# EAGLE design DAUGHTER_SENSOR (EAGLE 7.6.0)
DAUGHTER CARD SENSORS

## Sheet 1 of 3: HDK INTERFACE
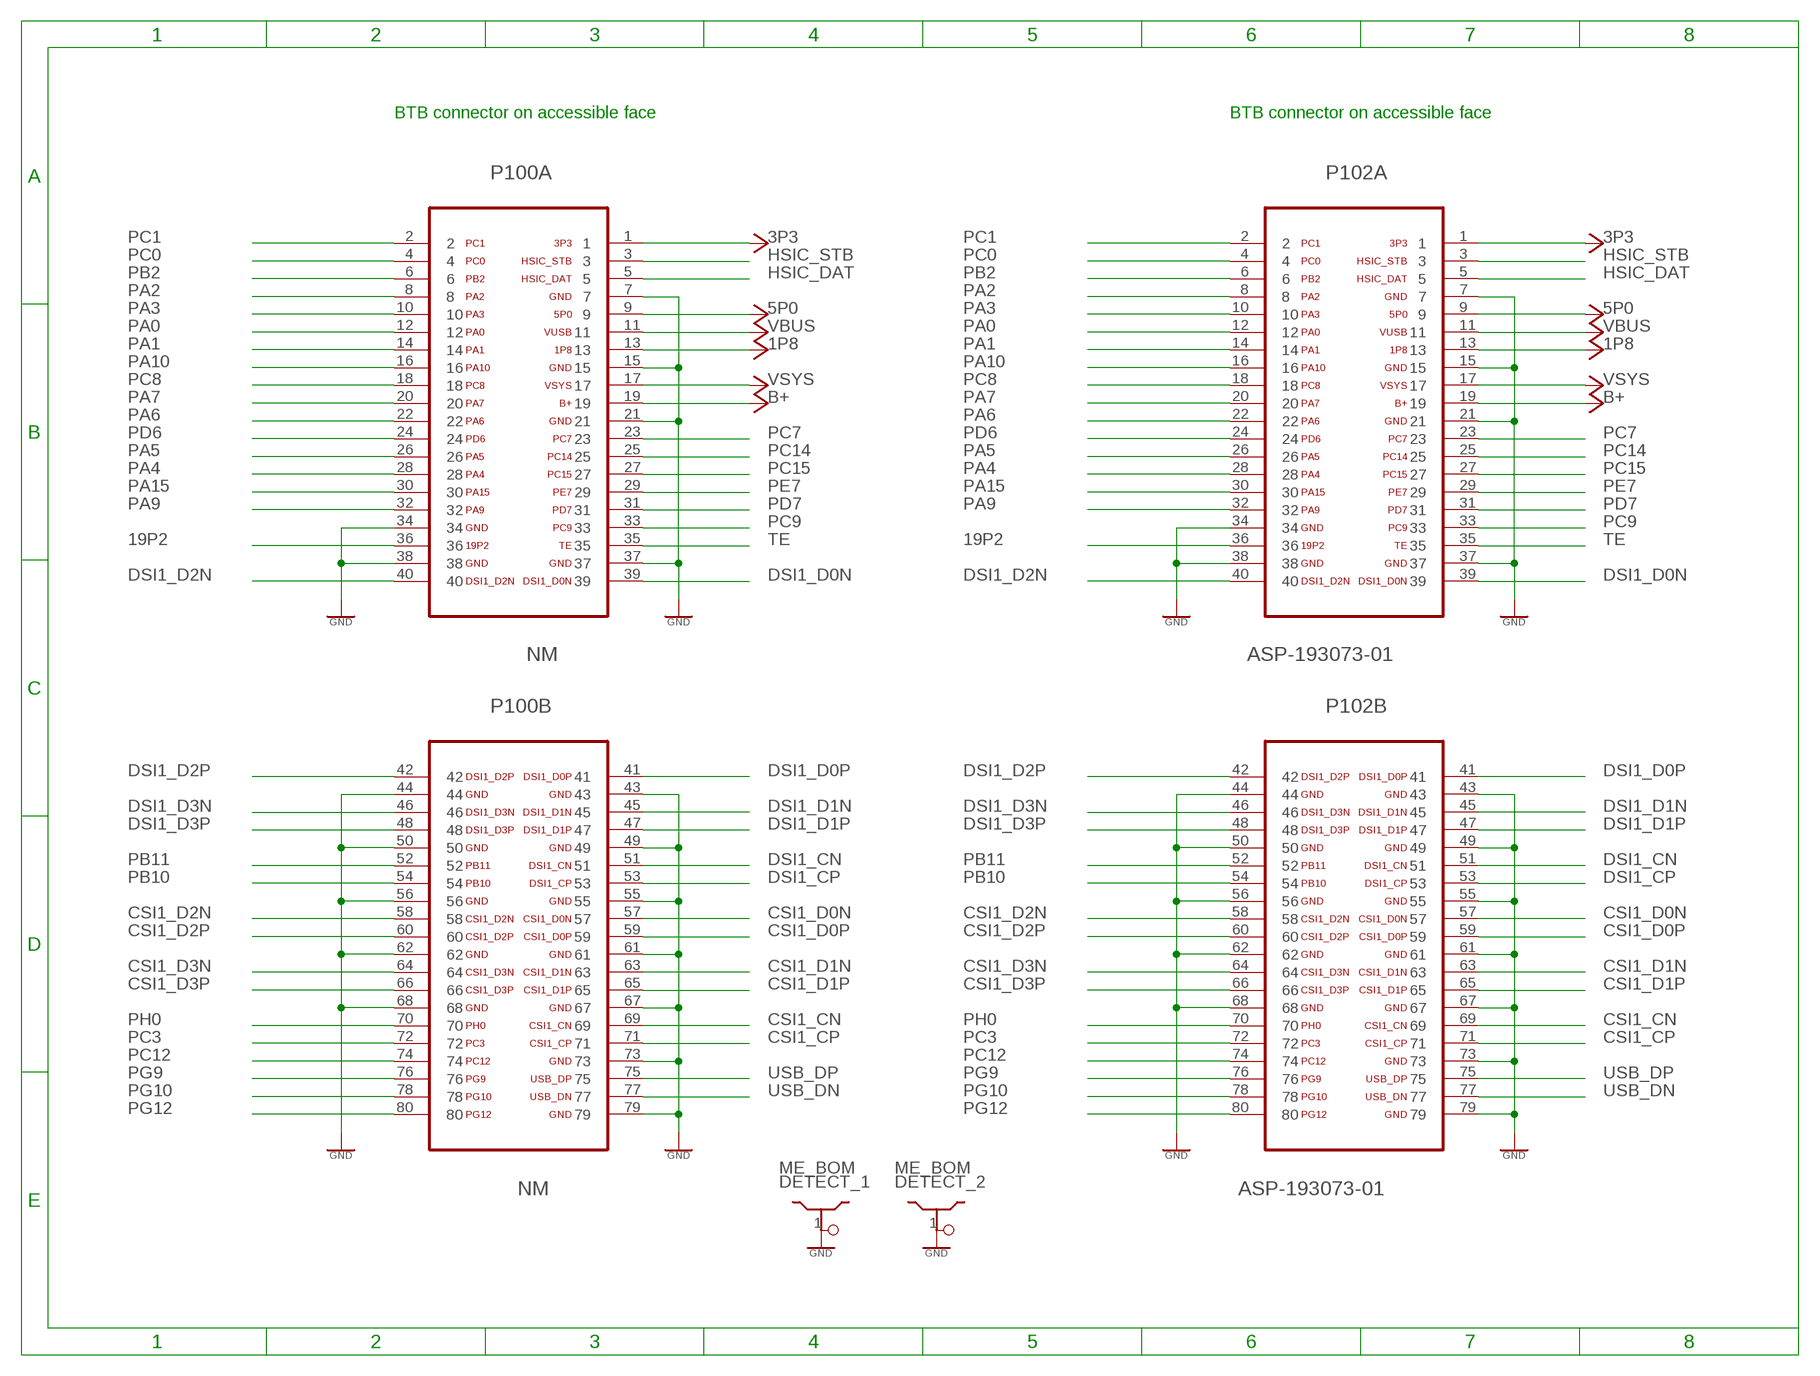
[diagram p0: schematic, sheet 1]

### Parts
DETECT_1  ME_BOM  SHIELDDETECT  [PLUG]
DETECT_2  ME_BOM  SHIELDDETECT  [PLUG]
P100  NM  CLM-140-02-L-D-KGOLD  [CLM-140-02-L-D-K_GOLD]
P102  ASP-193073-01  FTMH-140-02-L-DV-ES-P-TR  [FTMH-140-02-L-DV-ES-P-TR]

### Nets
1P8: P100.13 P102.13 ; also sheet 2,3
3P3: P100.1 P102.1 ; also sheet 2,3
5P0: P100.9 P102.9
19P2: P100.36 P102.36
B+: P100.19 P102.19
CSI1_CN: P100.69 P102.69
CSI1_CP: P100.71 P102.71
CSI1_D0N: P100.57 P102.57
CSI1_D0P: P100.59 P102.59
CSI1_D1N: P100.63 P102.63
CSI1_D1P: P100.65 P102.65
CSI1_D2N: P100.58 P102.58
CSI1_D2P: P100.60 P102.60
CSI1_D3N: P100.64 P102.64
CSI1_D3P: P100.66 P102.66
DSI1_CN: P100.51 P102.51
DSI1_CP: P100.53 P102.53
DSI1_D0N: P100.39 P102.39
DSI1_D0P: P100.41 P102.41
DSI1_D1N: P100.45 P102.45
DSI1_D1P: P100.47 P102.47
DSI1_D2N: P100.40 P102.40
DSI1_D2P: P100.42 P102.42
DSI1_D3N: P100.46 P102.46
DSI1_D3P: P100.48 P102.48
GND: DETECT_1.1 DETECT_2.1 P100.7 P100.15 P100.21 P100.34 P100.37 P100.38 P100.43 P100.44 P100.49 P100.50 P100.55 P100.56 P100.61 P100.62 P100.67 P100.68 P100.73 P100.79 P102.7 P102.15 P102.21 P102.34 P102.37 P102.38 P102.43 P102.44 P102.49 P102.50 P102.55 P102.56 P102.61 P102.62 P102.67 P102.68 P102.73 P102.79 ; also sheet 2,3
HSIC_DAT: P100.5 P102.5
HSIC_STB: P100.3 P102.3
PA0: P100.12 P102.12
PA1: P100.14 P102.14
PA2: P100.8 P102.8
PA3: P100.10 P102.10
PA4: P100.28 P102.28
PA5: P100.26 P102.26
PA6: P100.22 P102.22
PA7: P100.20 P102.20
PA9: P100.32 P102.32
PA10: P100.16 P102.16
PA15: P100.30 P102.30
PB2: P100.6 P102.6
PB10: P100.54 P102.54 ; also sheet 2
PB11: P100.52 P102.52 ; also sheet 2
PC0: P100.4 P102.4 ; also sheet 3
PC1: P100.2 P102.2 ; also sheet 3
PC3: P100.72 P102.72 ; also sheet 3
PC7: P100.23 P102.23
PC8: P100.18 P102.18
PC9: P100.33 P102.33
PC12: P100.74 P102.74
PC14: P100.25 P102.25
PC15: P100.27 P102.27
PD6: P100.24 P102.24
PD7: P100.31 P102.31
PE7: P100.29 P102.29
PG9: P100.76 P102.76 ; also sheet 2
PG10: P100.78 P102.78 ; also sheet 3
PG12: P100.80 P102.80
PH0: P100.70 P102.70
TE: P100.35 P102.35
USB_DN: P100.77 P102.77
USB_DP: P100.75 P102.75
VBUS: P100.11 P102.11
VSYS: P100.17 P102.17

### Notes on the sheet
- BTB connector on accessible face | BTB connector on accessible face

## Sheet 2 of 3: Identification
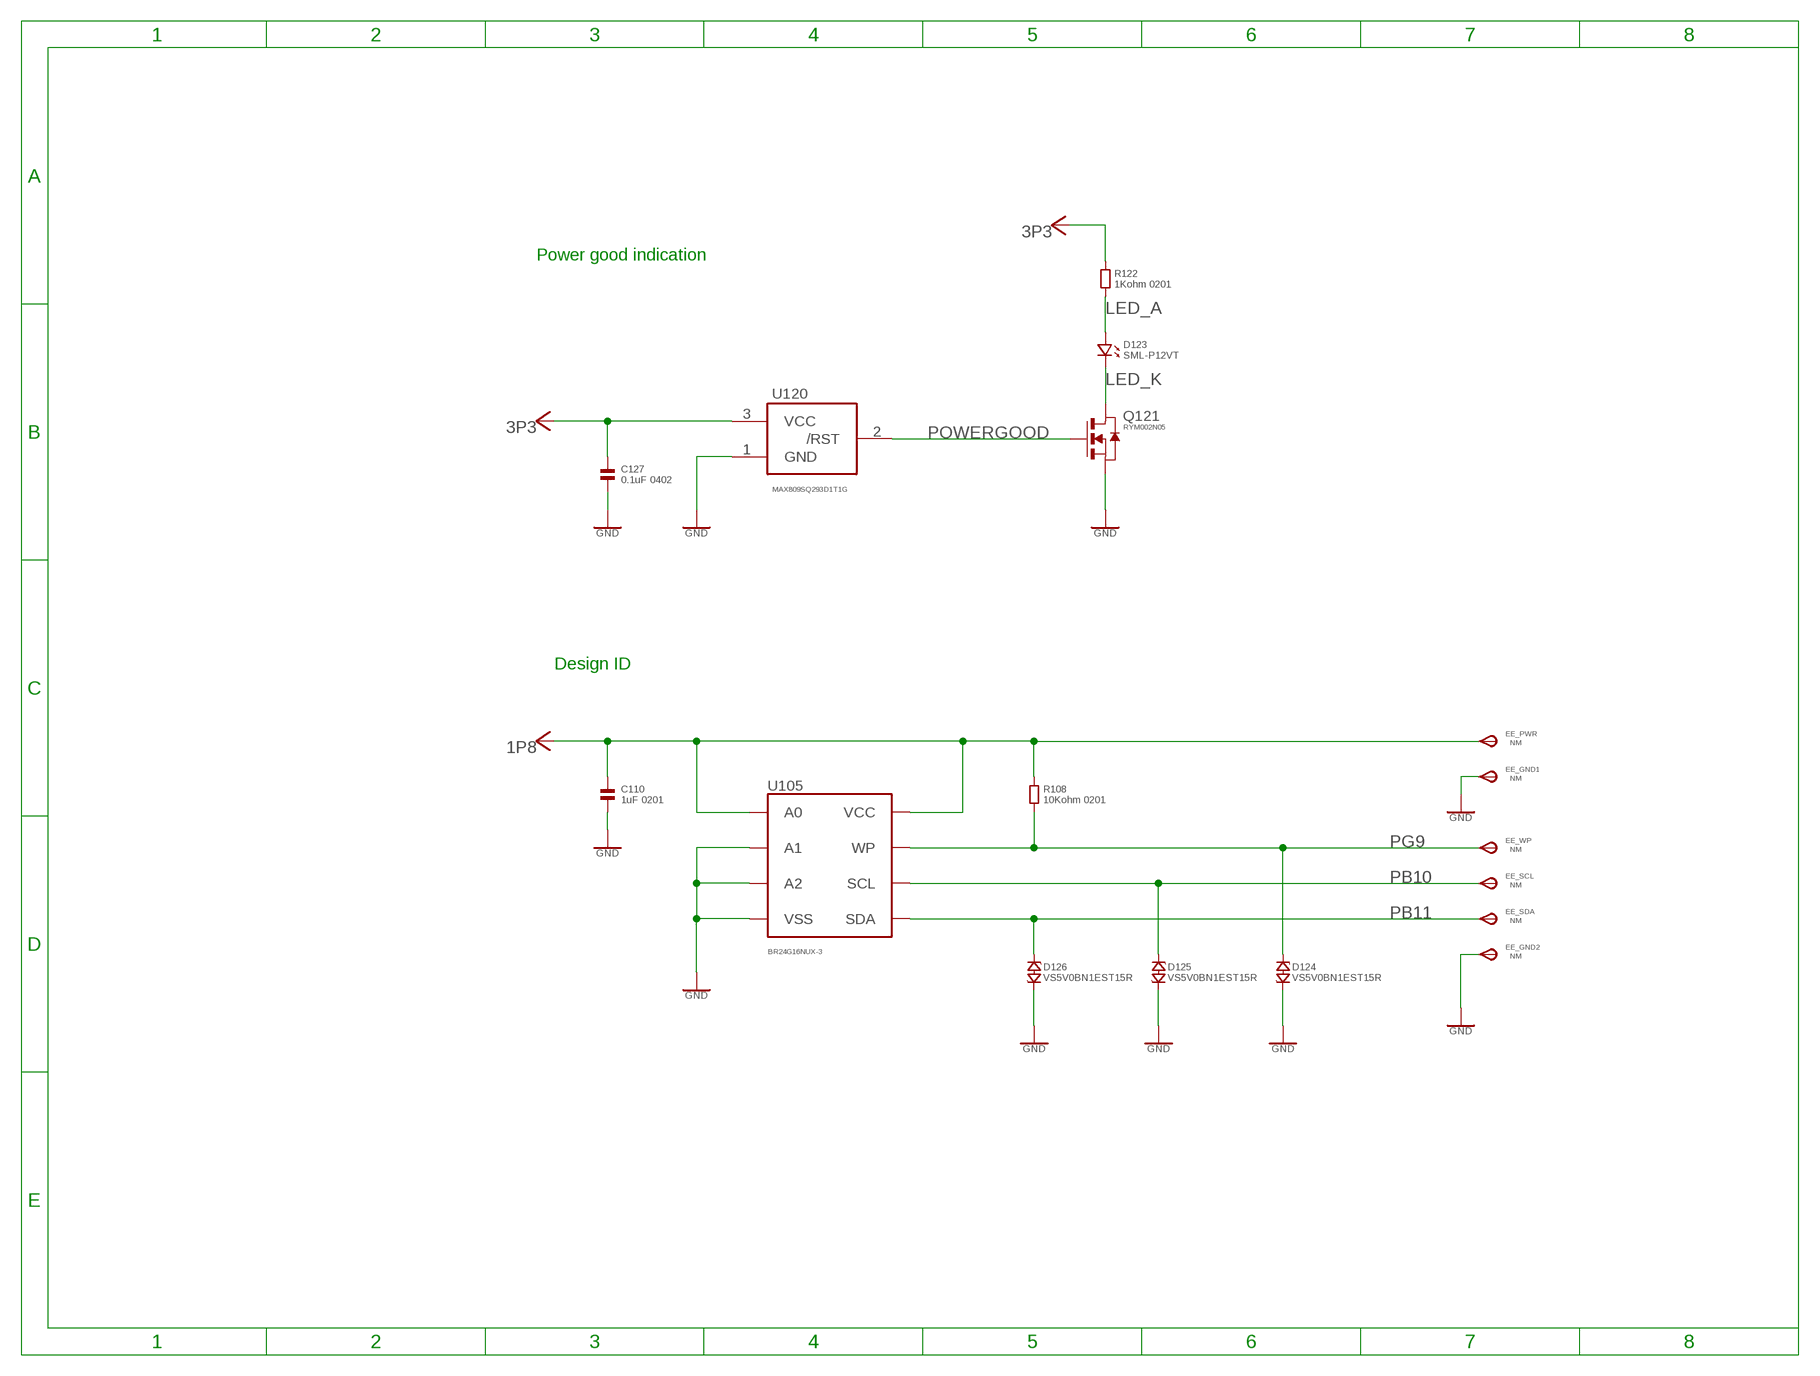
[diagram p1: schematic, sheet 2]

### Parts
C110  1uF 0201  CAPACITOR.0201  [0201]
C127  0.1uF 0402  CAPACITOR.0402  [0402]
D123  SML-P12VT  LED.0503  [0503.LED]
D124  VS5V0BN1EST15R  ESD_VARISTOR.0201  [CHIP_0201]
D125  VS5V0BN1EST15R  ESD_VARISTOR.0201  [CHIP_0201]
D126  VS5V0BN1EST15R  ESD_VARISTOR.0201  [CHIP_0201]
EE_GND1  NM  TPSTP11R  [TP11R]
EE_GND2  NM  TPSTP11R  [TP11R]
EE_PWR  NM  TPSTP11R  [TP11R]
EE_SCL  NM  TPSTP11R  [TP11R]
EE_SDA  NM  TPSTP11R  [TP11R]
EE_WP  NM  TPSTP11R  [TP11R]
Q121  RYM002N05  FET-NRYM002N05  [VMT3]
R108  10Kohm 0201  RESISTOR.0201  [0201]
R122  1Kohm 0201  RESISTOR.0201  [0201]
U105  BR24G16NUX-3  EEPROMDFN8  [DFN-8]
U120  MAX809SQ293D1T1G  MAX809  [SC70-3L]

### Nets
1P8: C110.1 EE_PWR.TP(PP) R108.1 U105.P$1(A0) U105.P$8(VCC) ; also sheet 1,3
3P3: C127.1 R122.1 U120.3(VCC) ; also sheet 1,3
GND: C110.2 C127.2 D124.P$2 D125.P$2 D126.P$2 EE_GND1.TP(PP) EE_GND2.TP(PP) Q121.2(S) U105.P$2(A1) U105.P$3(A2) U105.P$4(VSS) U105.P$9(VSS) U120.1(GND) ; also sheet 1,3
LED_A: D123.P$1 R122.2
LED_K: D123.P$2 Q121.3(D)
PB10: D125.P$1 EE_SCL.TP(PP) U105.P$6(SCL) ; also sheet 1
PB11: D126.P$1 EE_SDA.TP(PP) U105.P$5(SDA) ; also sheet 1
PG9: D124.P$1 EE_WP.TP(PP) R108.2 U105.P$7(WP) ; also sheet 1
POWERGOOD: Q121.1(G) U120.2(/RST)

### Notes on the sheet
- Power good indication
- Design ID

## Sheet 3 of 3: SENSOR
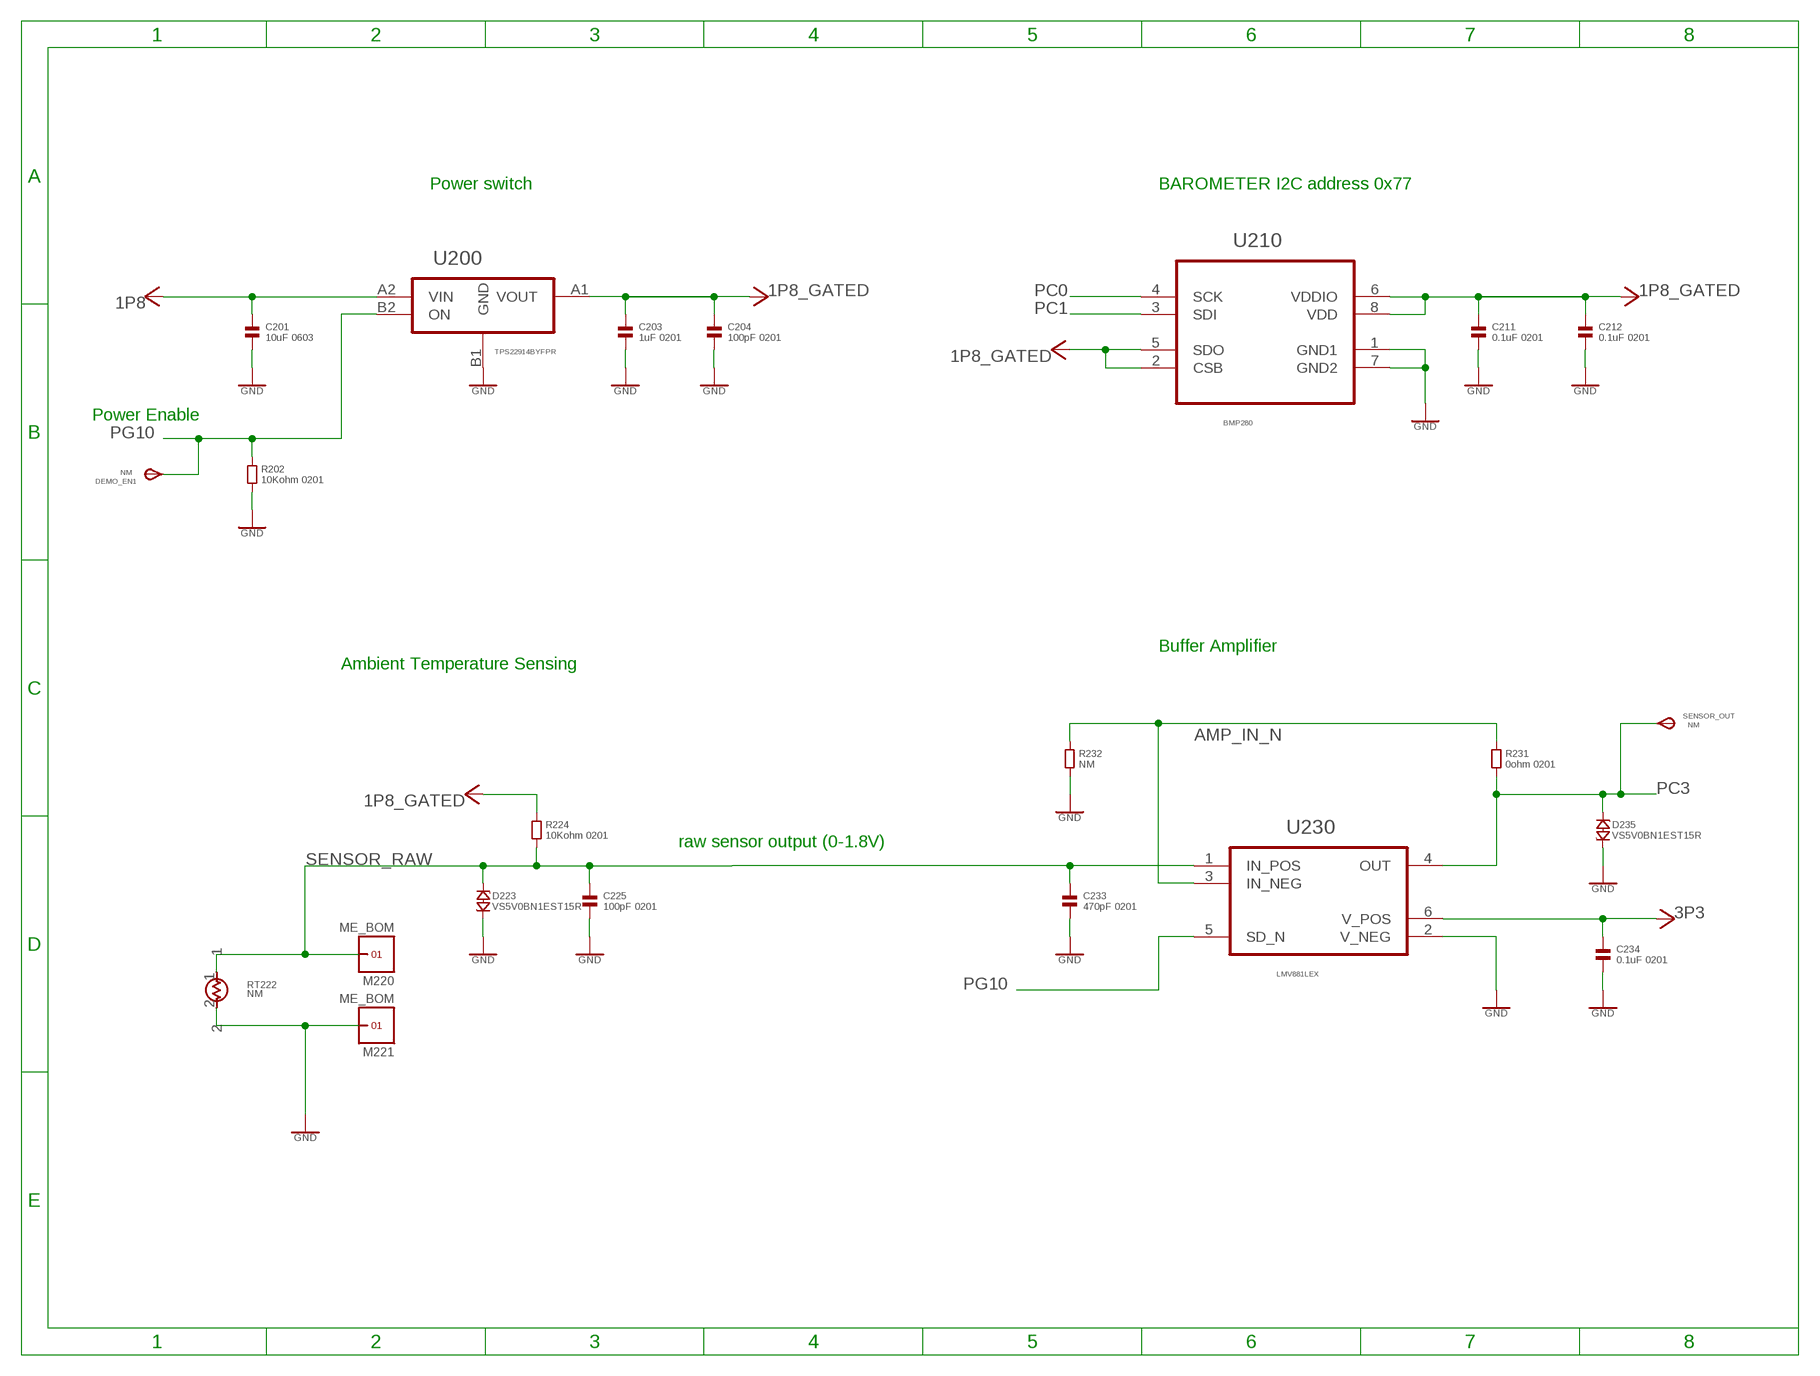
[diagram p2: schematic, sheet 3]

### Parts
C201  10uF 0603  CAPACITOR.0603  [0603]
C203  1uF 0201  CAPACITOR.0201  [0201]
C204  100pF 0201  CAPACITOR.0201  [0201]
C211  0.1uF 0201  CAPACITOR.0201  [0201]
C212  0.1uF 0201  CAPACITOR.0201  [0201]
C225  100pF 0201  CAPACITOR.0201  [0201]
C233  470pF 0201  CAPACITOR.0201  [0201]
C234  0.1uF 0201  CAPACITOR.0201  [0201]
D223  VS5V0BN1EST15R  ESD_VARISTOR.0201  [CHIP_0201]
D235  VS5V0BN1EST15R  ESD_VARISTOR.0201  [CHIP_0201]
DEMO_EN1  NM  TPSTP11R  [TP11R]
M220  ME_BOM  UNVERSA_CONTACT  [UNIVERSAL_CONTACT]
M221  ME_BOM  UNVERSA_CONTACT  [UNIVERSAL_CONTACT]
R202  10Kohm 0201  RESISTOR.0201  [0201]
R224  10Kohm 0201  RESISTOR.0201  [0201]
R231  0ohm 0201  RESISTOR.0201  [0201]
R232  NM  RESISTOR.0201  [0201]
RT222  NM  THERMISTOR  [0201]
SENSOR_OUT  NM  TPSTP11R  [TP11R]
U200  TPS22914BYFPR  [BGA0_75SQ_PS0_4_P4]
U210  BMP280  [LGA2X2_5PS0_65_P8]
U230  LMV881LEX  [DFN1_5X1PS0_5P6]

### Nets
1P8: C201.1 U200.A2(VIN) ; also sheet 1,2
1P8_GATED: C203.1 C204.1 C211.1 C212.1 R224.1 U200.A1(VOUT) U210.2(CSB) U210.5(SDO) U210.6(VDDIO) U210.8(VDD)
3P3: C234.1 U230.6(V_POS) ; also sheet 1,2
AMP_IN_N: R231.1 R232.1 U230.3(IN_NEG)
GND: C201.2 C203.2 C204.2 C211.2 C212.2 C225.2 C233.2 C234.2 D223.P$2 D235.P$2 M221.G1 R202.2 R232.2 RT222.2 U200.B1(GND) U210.1(GND1) U210.7(GND2) U230.2(V_NEG) ; also sheet 1,2
PC0: U210.4(SCK) ; also sheet 1
PC1: U210.3(SDI) ; also sheet 1
PC3: D235.P$1 R231.2 SENSOR_OUT.TP(PP) U230.4(OUT) ; also sheet 1
PG10: DEMO_EN1.TP(PP) R202.1 U200.B2(ON) U230.5(SD_N) ; also sheet 1
SENSOR_RAW: C225.1 C233.1 D223.P$1 M220.G1 R224.2 RT222.1 U230.1(IN_POS)

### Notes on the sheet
- Power switch | BAROMETER I2C address 0x77
- Power Enable
- Buffer Amplifier
- Ambient Temperature Sensing
- raw sensor output (0-1.8V)

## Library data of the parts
C110 C127 C201 C203 C204 C211 C212 C225 C233 C234 = MOTO_LIB:CAPACITOR: Ceramic Capacitor, Generic
D123 = MOTO_LIB:LED: LED GENERIC, single, 2 pin; MPN: SML-P12VT; SUPPLIER: ROHM
D124-D126 D223 D235 = MOTO_LIB:ESD_VARISTOR: GENERIC varistor,single, 2 pin; MPN: VS5V0BN1EST15R; SUPPLIER: ROHM
DEMO_EN1 EE_GND1 EE_GND2 EE_PWR EE_SCL EE_SDA EE_WP SENSOR_OUT = MOTO_LIB:TPS: TEST Point, 1mm diameter, gold
DETECT_1 DETECT_2 = MOTO_LIB:SHIELD: Shield, Custom; MPN: refer to ME BOM; SUPPLIER: ref to ME BOM
M220 M221 = MOTO_LIB:UNVERSA_CONTACT: Universal contact, Generic; MPN: refer to ME BOM; SUPPLIER: ref to ME BOM
P100 = MOTO_LIB:CLM-140-02-L-D-K: MICRO SOCKET, 1.0MM pitch, SMD, 2X40WAY, Female; MPN: CLM-140-02-L-D-K; SUPPLIER: SAMTEC
P102 = MOTO_LIB:FTMH-140-02-L-DV-ES-P-TR: MICRO SOCKET, 1.0MM, SMD, 2X40WAY, MALE; MPN: ASP-193073-01; SUPPLIER: SAMTEC
Q121 = MOTO_LIB:FET-N: Generic NMOS FET; MPN: RYM002N05; SUPPLIER: ROHM
R108 R122 R202 R224 R231 R232 = MOTO_LIB:RESISTOR: Resistor - Generic
RT222 = MOTO_LIB:THERMISTOR: Thmistor, NTC 10Khm 3%, 0201; MPN: NCP03XV103XV103E05RL/NTCG0603UH103HT; SUPPLIER: MURARA/TDK
U105 = MOTO_LIB:EEPROM: I2C EE PROM, 8 pin; MPN: BR24G16NUX-3; SUPPLIER: ROHM
U120 = MOTO_LIB:MAX809: 3-Pin Microprocessor Reset Circuit; MPN: MAX809SQ293D1T1; SUPPLIER: ON-SEMI
U200 = MOTO_LIB:TPS22914BYFPR: 5V load switch; MPN: TPS22914BYFPR; SUPPLIER: TI
U210 = MOTO_LIB:BMP280: BAROMETER BMP280; MPN: BMP280; SUPPLIER: BOSCH
U230 = MOTO_LIB:LMV881LEX: LOW NOISE OPAMP with Shutdown.; MPN: LMV881LEX; SUPPLIER: TI

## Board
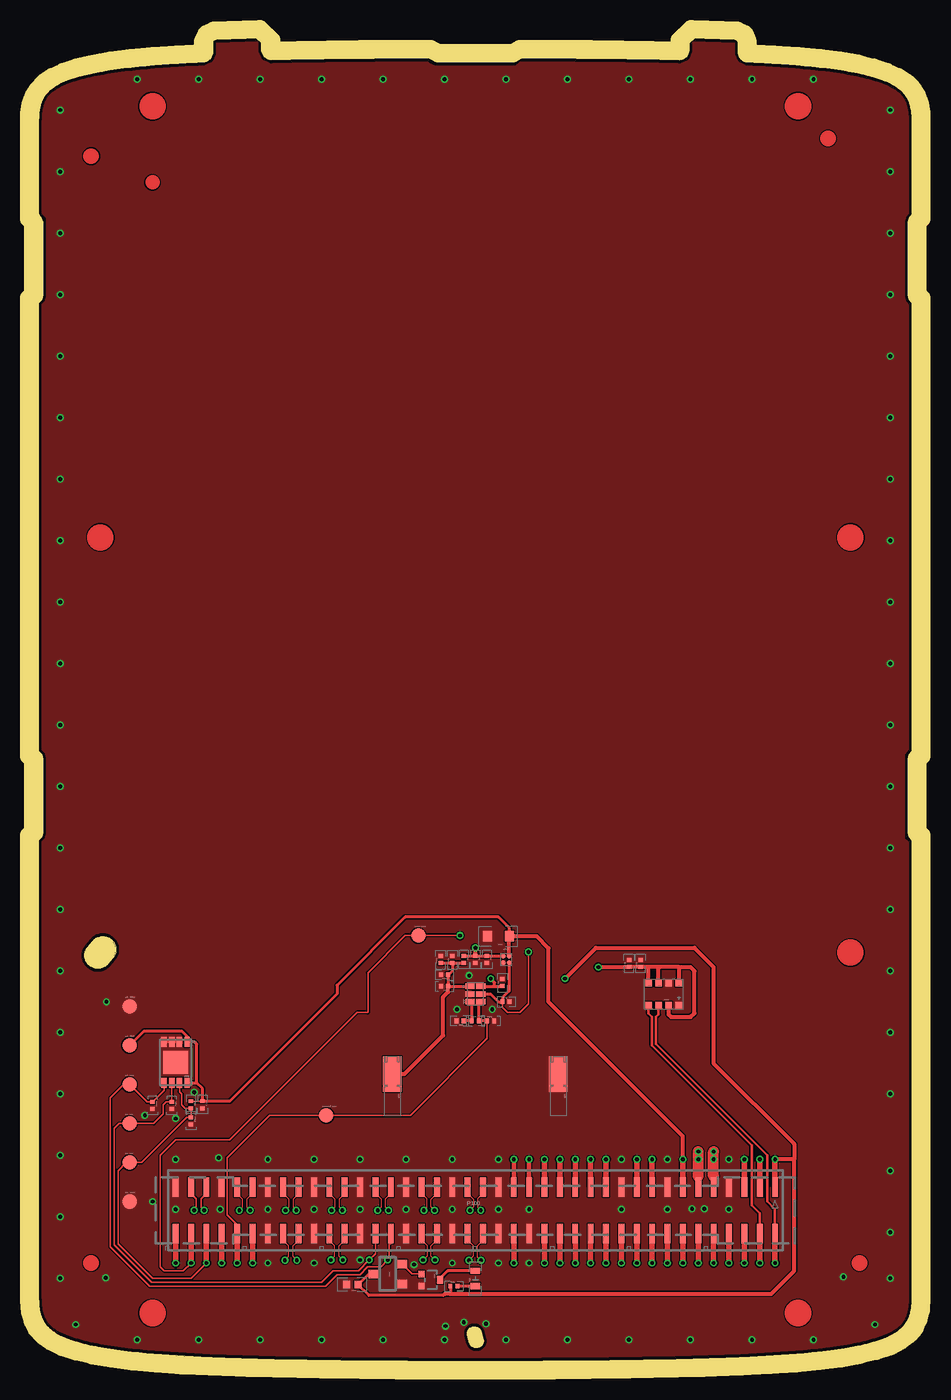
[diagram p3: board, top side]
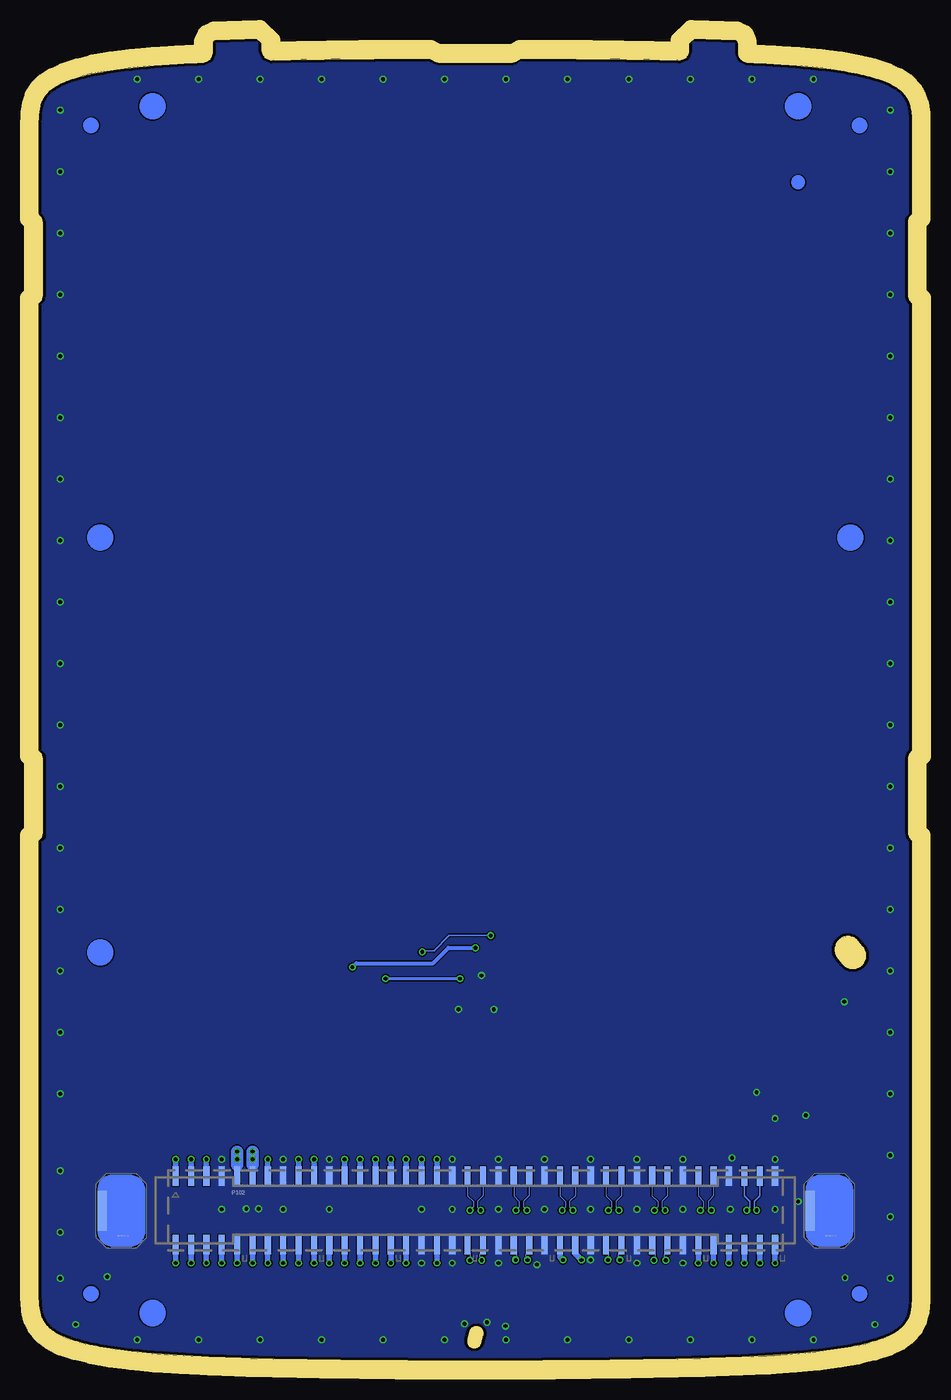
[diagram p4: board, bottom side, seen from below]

Size 56.85 x 86.03 mm. Coordinates in mm from the lower left corner, seen from the top.
Outline: 357 segments
Copper layers (1*2*15*16): Top 0.02mm / dielectric 0.045mm / Route2 0.016mm / dielectric 0.711mm / Route15 0.016mm / dielectric 0.045mm / Bottom 0.02mm
Design rules "constraint": minimum track width 0.08mm, minimum drill 0.25mm, track to track 0.08mm, track to pad 0.08mm, pad to pad 0.08mm, via to via 0.08mm, smd to smd 0.08mm, copper to edge 0.2mm, drill to drill 0.2mm, minimum pad ring 0.1mm, minimum via ring 0.1mm, stop-mask expansion 0mil, vias tented up to drill 0.25mm, thermal gap 0mil
Milling: 125 lines

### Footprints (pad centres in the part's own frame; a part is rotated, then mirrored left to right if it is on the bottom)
0201 = smd 0.25 x 0.3: 1 -0.23,0; 2 0.23,0
0402 = smd 0.45 x 0.5: 1 -0.37,0; 2 0.37,0
0603 = smd 0.58 x 0.68: 1 -0.71,0; 2 0.71,0
0503.LED = smd 0.4 x 0.6: P$1 -0.495,0; P$2 0.495,0
CHIP_0201 = smd 0.25 x 0.3: P$1 -0.23,0; P$2 0.23,0
TP11R = smd 0.95 x 0.95: TP 0,0
PLUG = smd 0.6 x 2.6: 1 -1.25,0
UNIVERSAL_CONTACT = smd 2.3 x 1.2: G1 -0.8,0
CLM-140-02-L-D-K_GOLD = smd 0.38 x 1.27: 1 19.5,1.52; 2 19.5,-1.52; 3 18.5,1.52; 4 18.5,-1.52; 5 17.5,1.52; 6 17.5,-1.52; 7 16.5,1.52; 8 16.5,-1.52; 9 15.5,1.52; 10 15.5,-1.52; 11 14.5,1.52; 12 14.5,-1.52; 13 13.5,1.52; 14 13.5,-1.52; 15 12.5,1.52; 16 12.5,-1.52; 17 11.5,1.52; 18 11.5,-1.52; 19 10.5,1.52; 20 10.5,-1.52; 21 9.5,1.52; 22 9.5,-1.52; 23 8.5,1.52; 24 8.5,-1.52; 25 7.5,1.52; 26 7.5,-1.52; 27 6.5,1.52; 28 6.5,-1.52; 29 5.5,1.52; 30 5.5,-1.52; 31 4.5,1.52; 32 4.5,-1.52; 33 3.5,1.52; 34 3.5,-1.52; 35 2.5,1.52; 36 2.5,-1.52; 37 1.5,1.52; 38 1.5,-1.52; 39 0.5,1.52; 40 0.5,-1.52; 41 -0.5,1.52; 42 -0.5,-1.52; 43 -1.5,1.52; 44 -1.5,-1.52; 45 -2.5,1.52; 46 -2.5,-1.52; 47 -3.5,1.52; 48 -3.5,-1.52; 49 -4.5,1.52; 50 -4.5,-1.52; 51 -5.5,1.52; 52 -5.5,-1.52; 53 -6.5,1.52; 54 -6.5,-1.52; 55 -7.5,1.52; 56 -7.5,-1.52; 57 -8.5,1.52; 58 -8.5,-1.52; 59 -9.5,1.52; 60 -9.5,-1.52; 61 -10.5,1.52; 62 -10.5,-1.52; 63 -11.5,1.52; 64 -11.5,-1.52; 65 -12.5,1.52; 66 -12.5,-1.52; 67 -13.5,1.52; 68 -13.5,-1.52; 69 -14.5,1.52; 70 -14.5,-1.52; 71 -15.5,1.52; 72 -15.5,-1.52; 73 -16.5,1.52; 74 -16.5,-1.52; 75 -17.5,1.52; 76 -17.5,-1.52; 77 -18.5,1.52; 78 -18.5,-1.52; 79 -19.5,1.52; 80 -19.5,-1.52
FTMH-140-02-L-DV-ES-P-TR = smd 0.4 x 1.263: 1 -19.5,2.223; 2 -19.5,-2.223; 3 -18.5,2.223; 4 -18.5,-2.223; 5 -17.5,2.223; 6 -17.5,-2.223; 7 -16.5,2.223; 8 -16.5,-2.223; 9 -15.5,2.223; 10 -15.5,-2.223; 11 -14.5,2.223; 12 -14.5,-2.223; 13 -13.5,2.223; 14 -13.5,-2.223; 15 -12.5,2.223; 16 -12.5,-2.223; 17 -11.5,2.223; 18 -11.5,-2.223; 19 -10.5,2.223; 20 -10.5,-2.223; 21 -9.5,2.223; 22 -9.5,-2.223; 23 -8.5,2.223; 24 -8.5,-2.223; 25 -7.5,2.223; 26 -7.5,-2.223; 27 -6.5,2.223; 28 -6.5,-2.223; 29 -5.5,2.223; 30 -5.5,-2.223; 31 -4.5,2.223; 32 -4.5,-2.223; 33 -3.5,2.223; 34 -3.5,-2.223; 35 -2.5,2.223; 36 -2.5,-2.223; 37 -1.5,2.223; 38 -1.5,-2.223; 39 -0.5,2.223; 40 -0.5,-2.223; 41 0.5,2.223; 42 0.5,-2.223; 43 1.5,2.223; 44 1.5,-2.223; 45 2.5,2.223; 46 2.5,-2.223; 47 3.5,2.223; 48 3.5,-2.223; 49 4.5,2.223; 50 4.5,-2.223; 51 5.5,2.223; 52 5.5,-2.223; 53 6.5,2.223; 54 6.5,-2.223; 55 7.5,2.223; 56 7.5,-2.223; 57 8.5,2.223; 58 8.5,-2.223; 59 9.5,2.223; 60 9.5,-2.223; 61 10.5,2.223; 62 10.5,-2.223; 63 11.5,2.223; 64 11.5,-2.223; 65 12.5,2.223; 66 12.5,-2.223; 67 13.5,2.223; 68 13.5,-2.223; 69 14.5,2.223; 70 14.5,-2.223; 71 15.5,2.223; 72 15.5,-2.223; 73 16.5,2.223; 74 16.5,-2.223; 75 17.5,2.223; 76 17.5,-2.223; 77 18.5,2.223; 78 18.5,-2.223; 79 19.5,2.223; 80 19.5,-2.223
VMT3 = smd 0.42 x 0.4: 1 -0.4,-0.6; 2 0.4,-0.6 | smd 0.52 x 0.4: 3 0,0.6
DFN-8 = smd 0.35 x 0.65: P$1 -0.75,-1.325; P$2 -0.25,-1.325; P$3 0.25,-1.325; P$4 0.75,-1.325; P$5 0.75,1.325; P$6 0.25,1.325; P$7 -0.25,1.325; P$8 -0.75,1.325 | smd 1.6 x 1.5: P$9 0,0
SC70-3L = smd 0.55 x 0.63: 1 -0.65,-0.94; 3 0,0.94 | smd 0.555 x 0.63: 2 0.65,-0.94
BGA0_75SQ_PS0_4_P4 = smd 0.32 x 0.32: A1 -0.2,0.2; A2 0.2,0.2; B1 -0.2,-0.2; B2 0.2,-0.2
LGA2X2_5PS0_65_P8 = smd 0.45 x 0.45: 1 -0.975,0.725; 2 -0.325,0.725; 3 0.325,0.725; 4 0.975,0.725; 5 0.975,-0.725; 6 0.325,-0.725; 7 -0.325,-0.725; 8 -0.975,-0.725
DFN1_5X1PS0_5P6 = smd 0.35 x 0.6: 1 0.5,0.35; 2 0,0.35; 3 -0.5,0.35; 4 -0.5,-0.35; 5 0,-0.35; 6 0.5,-0.35

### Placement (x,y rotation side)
C110  10.67,16.67 270 top
C127  20.42,4.97 180 top
C201  29.92,27.62 180 top
C203  29.17,26.12 270 top
C204  28.42,26.12 270 top
C211  39.17,25.87 90 top
C212  38.42,25.87 90 top
C225  26.17,26.12 90 top
C233  26.92,26.12 90 top
C234  30.17,24.62 90 top
D123  28.42,5.37 90 top
D124  9.92,15.62 270 top
D125  8.67,16.62 270 top
D126  7.42,16.62 270 top
D223  26.42,24.37 180 top
D235  29.42,22.12 0 top
DEMO_EN1  24.72,27.67 0 top
DETECT_1  51.45,9.77 0 bottom
DETECT_2  5.39,9.77 0 bottom
EE_GND1  5.92,10.37 0 top
EE_GND2  5.92,23.07 0 top
EE_PWR  5.92,20.53 0 top
EE_SCL  5.92,15.45 0 top
EE_SDA  5.92,17.99 0 top
EE_WP  5.92,12.91 0 top
M220  23.02,17.87 270 top
M221  33.82,17.87 270 top
P100  28.42,9.8 0 top
P102  28.42,9.8 0 bottom
Q121  25.52,5.27 270 top
R108  9.92,16.67 270 top
R122  27.02,4.87 0 top
R202  30.42,23.37 0 top
R224  27.67,26.12 270 top
R231  28.42,22.12 0 top
R232  27.42,22.12 180 top
RT222  26.42,25.12 180 top
SENSOR_OUT  18.72,15.97 0 top
U105  8.92,19.42 180 top
U120  22.72,5.67 90 top
U200  30.42,26.12 0 top
U210  40.67,23.87 180 top
U230  28.42,23.87 90 top

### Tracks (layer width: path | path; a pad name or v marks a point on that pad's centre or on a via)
1P8  (via drill 0.25)
  Top 0.1: R108.1 C110.1
  Top 0.2: EE_PWR.TP 6.86,21.47 9.32,21.47 9.67,21.12 U105.P$1 10.15,20.75 10.3,20.6 10.3,18.1 | U105.P$8 10.3,18.1 | 10.3,18.1 10.67,17.72 C110.1 12.45,16.9 19.42,23.87 19.42,24.44 23.86,28.87 29.92,28.87 30.63,28.16 C201.1
  Top 0.25: C201.1 32.42,27.62 33.19,26.86 33.19,23.36 41.92,14.62 v41.92,13.12 | U200.A2 C201.1
  Top 0.35: C201.1 | P100.13 v41.92,13.12
  Bottom 0.35: P102.13 v41.92,13.12
1P8_GATED  (via drill 0.25)
  Top 0.2: U200.A1 30.19,26.35 C203.1 C204.1 R224.1
  Top 0.25: C204.1 v28.42,26.87 | v36.42,25.62 38.4,25.62 C212.1 C211.1 39.19,25.62 39.67,25.62 | 41.65,25.62 41.65,24.62 U210.8 | U210.2 41,22.55 41.17,22.37 42.42,22.37 42.67,22.62 42.67,25.37 | 42.67,25.37 42.42,25.62 | 42.42,25.62 42.67,25.37 | 41.65,25.62 41.67,25.62 42.42,25.62 | 41.65,25.62 40.42,25.62 | 40.42,25.62 39.67,25.62 | U210.6 40.35,25.55 40.42,25.62 | U210.5 39.7,25.6 39.67,25.62
  Bottom 0.25: v28.42,26.87 30.17,26.87 31.17,25.87 36.17,25.87 v36.42,25.62
3P3  (via drill 0.25)
  Top 0.2: U230.6 29.67,24.37 | 29.67,24.37 30.15,24.37 C234.1 | 29.67,24.37 29.67,24.62 v29.42,24.87 | U120.3 21.49,5.67 C127.1 21.49,4.27 26.32,4.27 26.42,4.37 | R122.1 26.79,4.37
  Top 0.25: v34.26,24.87 36.26,26.87 42.67,26.87 43.92,25.62 43.92,19.37 49.17,14.12 49.17,13.12 | 49.17,13.12 v47.92,13.12 | 26.42,4.37 26.79,4.37 47.67,4.37 49.17,5.87 49.17,13.12
  Top 0.35: P100.1 v47.92,13.12
  Bottom 0.2: v29.42,24.87 v34.26,24.87
  Bottom 0.35: P102.1 v47.92,13.12
5P0  (via drill 0.25)
  Top 0.25: P100.9 P102.9
  Top 0.7: P102.9 v43.92,13.62
  Bottom 0.4: P102.9 43.92,12.77
  Bottom 0.8: 43.92,12.77 v43.92,13.12 v43.92,13.62
19P2  (via drill 0.25)
  Top 0.35: P100.36 v30.92,6.37
  Bottom 0.35: v30.92,6.37 P102.36
AMP_IN_N
  Top 0.2: R232.1 R231.1 28.19,23.25 U230.3
B+  (via drill 0.25)
  Top 0.35: P100.19 v38.92,13.12
  Bottom 0.35: v38.92,13.12 P102.19
CSI1_CN  (via drill 0.25)
  Top 0.08: P100.69 13.92,10.9 13.57,10.55 13.57,10 v13.77,9.8
  Bottom 0.08: P102.69 13.92,10.75 13.57,10.4 13.57,10 v13.77,9.8
CSI1_CP  (via drill 0.25)
  Top 0.08: P100.71 12.92,10.9 13.29,10.53 13.29,10.02 v13.07,9.8
  Bottom 0.08: P102.71 12.92,10.75 13.27,10.4 13.27,10 v13.07,9.8
CSI1_D0N  (via drill 0.25)
  Top 0.08: P100.57 19.92,10.9 19.55,10.53 19.55,10.02 v19.77,9.8
  Bottom 0.08: P102.57 19.92,10.75 19.57,10.4 19.57,10 v19.77,9.8
CSI1_D0P  (via drill 0.25)
  Top 0.08: P100.59 18.92,10.9 19.27,10.55 19.27,10 v19.07,9.8
  Bottom 0.08: P102.59 18.92,10.75 19.29,10.38 19.29,10.02 v19.07,9.8
CSI1_D1N  (via drill 0.25)
  Top 0.08: P100.63 16.92,10.9 16.55,10.53 16.55,10.02 v16.77,9.8
  Bottom 0.08: P102.63 16.92,10.75 16.55,10.38 16.55,10.02 v16.77,9.8
CSI1_D1P  (via drill 0.25)
  Top 0.08: 15.92,10.9 16.27,10.55 16.27,10 v16.07,9.8
  Top 0.1: P100.65 15.92,10.9
  Bottom 0.08: P102.65 15.92,10.75 16.27,10.4 16.27,10 v16.07,9.8
CSI1_D2N  (via drill 0.25)
  Top 0.08: P100.58 19.92,7.85 19.57,7.5 19.57,6.8 v19.8,6.58
  Bottom 0.08: P102.58 19.92,7.17 19.72,6.97 19.72,6.65 v19.8,6.58
CSI1_D2P  (via drill 0.25)
  Top 0.08: P100.60 18.92,7.85 19.27,7.5 19.27,6.82 v19.03,6.58
  Bottom 0.08: P102.60 18.92,7.15 19.12,6.95 19.12,6.67 v19.03,6.58
CSI1_D3N  (via drill 0.25)
  Top 0.08: P100.64 16.92,7.85 16.57,7.5 16.57,6.8 v16.81,6.57
  Bottom 0.08: P102.64 16.92,7.12 16.72,6.92 16.72,6.65 v16.81,6.57
CSI1_D3P  (via drill 0.25)
  Top 0.08: P100.66 15.92,7.85 16.27,7.5 16.27,6.8 v16.03,6.57
  Bottom 0.08: P102.66 15.92,7.12 16.12,6.92 16.12,6.65 v16.03,6.57
DSI1_CN  (via drill 0.25)
  Top 0.08: 22.92,10.9 22.55,10.53 22.55,10.02 v22.77,9.8
  Top 0.1: P100.51 22.92,10.9
  Bottom 0.08: P102.51 22.92,10.75 22.57,10.4 22.57,10 v22.77,9.8
DSI1_CP  (via drill 0.25)
  Top 0.08: P100.53 21.92,10.9 22.27,10.55 22.27,10 v22.07,9.8
  Bottom 0.08: P102.53 21.92,10.75 22.29,10.39 22.29,10.02 v22.07,9.8
DSI1_D0N  (via drill 0.25)
  Top 0.08: P100.39 28.92,10.9 28.57,10.55 28.57,10 v28.77,9.8
  Bottom 0.08: P102.39 28.92,10.75 28.55,10.38 28.55,10.02 v28.77,9.8
DSI1_D0P  (via drill 0.25)
  Top 0.08: P100.41 27.92,10.9 28.29,10.53 28.29,10.02 v28.07,9.8
  Bottom 0.08: P102.41 27.92,10.75 28.27,10.4 28.27,10 v28.07,9.8
DSI1_D1N  (via drill 0.25)
  Top 0.08: P100.45 25.92,10.9 25.55,10.53 25.55,10.02 v25.77,9.8
  Bottom 0.08: P102.45 25.92,10.75 25.57,10.4 25.57,10 v25.77,9.8
DSI1_D1P  (via drill 0.25)
  Top 0.08: P100.47 24.92,10.9 25.27,10.55 25.27,10 v25.07,9.8
  Bottom 0.08: P102.47 24.92,10.75 25.29,10.38 25.29,10.02 v25.07,9.8
DSI1_D2N  (via drill 0.25)
  Top 0.08: P100.40 28.92,7.85 28.57,7.5 28.57,6.76 v28.78,6.56
  Bottom 0.08: P102.40 28.92,7.17 28.72,6.97 28.72,6.61 v28.78,6.56
DSI1_D2P  (via drill 0.25)
  Top 0.08: P100.42 27.92,7.85 28.29,7.48 28.29,6.84 v28.01,6.56
  Bottom 0.08: P102.42 27.92,7.15 28.12,6.95 28.12,6.67 v28.01,6.56
DSI1_D3N  (via drill 0.25)
  Top 0.08: P100.46 25.92,7.87 25.56,7.5 25.55,6.82 v25.8,6.58
  Bottom 0.08: P102.46 25.92,7.17 25.72,6.97 25.72,6.65 v25.8,6.58
DSI1_D3P  (via drill 0.25)
  Top 0.08: P100.48 24.92,7.87 25.27,7.52 25.27,6.82 v25.03,6.58
  Bottom 0.08: P102.48 24.92,7.15 25.12,6.95 25.12,6.67 v25.03,6.58
GND  (via drill 0.25)
  Top 0.2: U105.P$4 U105.P$3 U105.P$2
  other vias: 14.42,1.37 10.42,1.37 6.42,1.37 22.42,1.37 18.42,1.37 26.42,1.37 30.42,1.37 34.42,1.37 38.42,1.37 42.42,1.37 46.42,1.37 50.42,1.37 54.42,2.37 55.42,8.37 55.42,5.37 55.42,12.37 55.42,17.37 55.42,21.37 55.42,25.37 55.42,29.37 55.42,33.37 55.42,37.37 55.42,41.37 55.42,45.37 55.42,49.37 55.42,53.37 55.42,57.37 55.42,61.37 55.42,65.37 55.42,69.37 55.42,73.37 55.42,77.37 55.42,81.37 50.42,83.37 46.42,83.37 42.42,83.37 38.42,83.37 34.42,83.37 30.42,83.37 26.42,83.37 22.42,83.37 18.42,83.37 14.42,83.37 10.42,83.37 6.42,83.37 1.42,81.37 1.42,77.37 1.42,73.37 1.42,69.37 1.42,65.37 1.42,61.37 1.42,57.37 1.42,53.37 1.42,49.37 1.42,45.37 1.42,41.37 1.42,37.37 1.42,33.37 1.42,29.37 1.42,25.37 4.42,23.37 1.42,21.37 1.42,17.37 1.42,13.37 1.42,9.37 1.42,5.37 2.42,2.37 8.92,13.12 11.72,13.22 14.92,13.12 17.92,13.12 20.92,13.12 23.92,13.12 26.92,13.12 29.92,13.12 29.92,9.87 31.92,9.87 26.92,9.87 23.92,9.87 20.92,9.87 17.92,9.87 14.92,9.87 11.82,9.87 8.92,9.87 7.42,10.37 8.92,15.77 10.12,17.47 14.92,6.37 17.92,6.37 20.92,6.57 24.42,6.27 26.92,6.37 29.92,6.37 31.92,6.37 44.92,9.87 42.52,9.9 43.32,9.9 40.92,9.87 37.92,9.87 37.92,13.12 40.92,13.12 44.92,13.12 29.52,22.87 28.02,25.07 27.22,22.87 6.92,15.97 29.12,2.42 27.67,2.52 26.47,2.27 52.37,5.47 4.37,5.42
  pour Top: 25.82,84.22 31.07,84.22 31.57,84.67 36.72,84.67 41.82,84.57 42.12,84.67 42.32,84.97 42.42,85.17 42.42,85.57 42.72,85.97 45.32,85.87 45.42,85.67 45.42,84.97 45.62,84.57 45.82,84.47 46.12,84.37 47.12,84.37 50.02,84.17 51.72,83.97 53.32,83.67 54.82,83.27 55.72,82.87 56.22,82.47 56.52,82.07 56.72,81.47 56.82,80.77 56.82,74.97 56.42,74.47 56.32,74.07 56.32,69.27 56.42,68.87 56.82,68.47 56.82,39.97 56.32,39.47 56.32,33.97 56.82,33.57 56.82,4.87 56.72,3.47 56.52,2.67 56.12,2.17 55.52,1.77 54.22,1.27 52.92,0.97 51.62,0.77 48.72,0.47 44.72,0.27 43.62,0.27 43.32,0.37 38.32,0.27 38.02,0.17 36.62,0.07 20.12,0.07 18.72,0.17 18.52,0.27 13.52,0.37 13.22,0.27 10.82,0.37 7.02,0.57 3.92,0.97 2.32,1.37 1.32,1.77 0.72,2.17 0.42,2.47 0.22,2.97 0.12,3.47 0.02,4.47 0.02,33.57 0.42,33.97 0.52,34.27 0.52,39.27 0.32,39.67 0.12,39.97 0.02,40.07 0.02,68.47 0.32,68.77 0.52,69.17 0.52,74.37 0.02,74.87 0.02,80.27 0.12,81.27 0.42,82.27 0.72,82.57 1.72,83.17 3.02,83.57 4.52,83.87 7.02,84.17 9.92,84.37 10.82,84.37 11.22,84.57 11.42,84.87 11.42,85.67 11.52,85.87 14.12,85.97 14.42,85.67 14.42,85.07 14.62,84.77 14.92,84.57 15.52,84.57 19.92,84.67 25.17,84.67 25.37,84.42
  pour Bottom: 25.82,84.27 31.02,84.27 31.42,84.47 31.62,84.67 36.72,84.67 41.82,84.57 42.12,84.67 42.32,84.97 42.42,85.17 42.42,85.57 42.72,85.97 45.32,85.87 45.42,85.67 45.42,84.97 45.62,84.57 45.82,84.47 46.12,84.37 47.12,84.37 50.02,84.17 51.72,83.97 53.32,83.67 54.82,83.27 55.72,82.87 56.22,82.47 56.52,82.07 56.72,81.47 56.82,80.77 56.82,74.97 56.42,74.47 56.32,74.07 56.32,69.27 56.42,68.87 56.82,68.47 56.82,39.97 56.32,39.47 56.32,33.97 56.82,33.57 56.82,4.87 56.72,3.47 56.52,2.67 56.12,2.17 55.52,1.77 54.22,1.27 52.92,0.97 51.62,0.77 48.72,0.47 44.72,0.27 43.62,0.27 43.32,0.37 38.32,0.27 38.02,0.17 36.62,0.07 20.12,0.07 18.72,0.17 18.52,0.27 13.52,0.37 13.22,0.27 10.82,0.37 7.02,0.57 3.92,0.97 2.32,1.37 1.32,1.77 0.72,2.17 0.42,2.47 0.22,2.97 0.12,3.47 0.02,4.47 0.02,33.57 0.42,33.97 0.52,34.27 0.52,39.27 0.32,39.67 0.12,39.97 0.02,40.07 0.02,68.47 0.32,68.77 0.52,69.17 0.52,74.37 0.02,74.87 0.02,80.27 0.12,81.27 0.42,82.27 0.72,82.57 1.72,83.17 3.02,83.57 4.52,83.87 7.02,84.17 9.92,84.37 10.82,84.37 11.22,84.57 11.42,84.87 11.42,85.67 11.52,85.87 14.12,85.97 14.42,85.67 14.42,85.07 14.62,84.77 14.92,84.57 15.52,84.57 19.92,84.67 25.32,84.67 25.62,84.37
HSIC_DAT  (via drill 0.25)
  Top 0.35: P100.5 v45.92,13.12
  Bottom 0.35: v45.92,13.12 P102.5
HSIC_STB  (via drill 0.25)
  Top 0.35: P100.3 v46.92,13.12
  Bottom 0.35: v46.92,13.12 P102.3
LED_A
  Top 0.1: R122.2
  Top 0.2: D123.P$1 R122.2
LED_K
  Top 0.2: D123.P$2 26.62,5.87 26.22,5.47 26.22,5.37 Q121.3
PA0  (via drill 0.25)
  Top 0.35: P100.12 v42.92,6.37
  Bottom 0.35: v42.92,6.37 P102.12
PA1  (via drill 0.25)
  Top 0.35: P100.14 v41.92,6.37
  Bottom 0.35: v41.92,6.37 P102.14
PA2  (via drill 0.25)
  Top 0.35: P100.8 v44.92,6.37
  Bottom 0.35: v44.92,6.37 P102.8
PA3  (via drill 0.25)
  Top 0.35: P100.10 v43.92,6.37
  Bottom 0.35: v43.92,6.37 P102.10
PA4  (via drill 0.25)
  Top 0.35: P100.28 v34.92,6.37
  Bottom 0.35: v34.92,6.37 P102.28
PA5  (via drill 0.25)
  Top 0.35: P100.26 v35.92,6.37
  Bottom 0.35: v35.92,6.37 P102.26
PA6  (via drill 0.25)
  Top 0.35: P100.22 v37.92,6.37
  Bottom 0.35: v37.92,6.37 P102.22
PA7  (via drill 0.25)
  Top 0.35: P100.20 v38.92,6.37
  Bottom 0.35: v38.92,6.37 P102.20
PA9  (via drill 0.25)
  Top 0.35: P100.32 v32.92,6.37
  Bottom 0.35: v32.92,6.37 P102.32
PA10  (via drill 0.25)
  Top 0.35: P100.16 v40.92,6.37
  Bottom 0.35: v40.92,6.37 P102.16
PA15  (via drill 0.25)
  Top 0.35: P100.30 v33.92,6.37
  Bottom 0.35: v33.92,6.37 P102.30
PB2  (via drill 0.25)
  Top 0.35: P100.6 v45.92,6.37
  Bottom 0.35: v45.92,6.37 P102.6
PB10  (via drill 0.25)
  Top 0.1: P100.54 21.92,6.97 v21.52,6.57 20.82,5.87 19.17,5.87 18.42,5.12 7.37,5.12 4.92,7.57 4.92,15.12 5.25,15.45 EE_SCL.TP 7.5,15.45 8.12,16.07 8.12,16.67 8.3,16.85 D125.P$1 U105.P$6
  Bottom 0.35: P102.54 21.92,6.97 v21.52,6.57
PB11  (via drill 0.25)
  Top 0.1: P100.52 22.92,7.67 22.82,7.57 22.82,6.67 v22.72,6.57 22.27,6.12 21.42,6.12 20.92,5.62 19.42,5.62 18.67,4.87 7.22,4.87 4.67,7.42 4.67,17.12 5.54,17.99 EE_SDA.TP 7.06,16.85 D126.P$1 8.17,17.6 U105.P$5
  Bottom 0.35: P102.52 22.92,6.77 v22.72,6.57
PC0  (via drill 0.25)
  Top 0.15: P100.4 46.92,9.62 46.42,10.12 46.42,14.02 39.92,20.52 39.92,22.37 39.7,22.6 U210.4
  Top 0.35: P100.4 v46.92,6.37
  Bottom 0.35: P102.4 v46.92,6.37
PC1  (via drill 0.25)
  Top 0.15: U210.3 40.35,22.55 40.17,22.37 40.17,20.62 47.42,13.37 47.42,10.37 47.92,9.87 P100.2
  Top 0.35: P100.2 v47.92,6.37
  Bottom 0.35: P102.2 v47.92,6.37
PC3  (via drill 0.25)
  Top 0.1: D235.P$1 29.19,20.97 24.19,15.97 SENSOR_OUT.TP 15.02,15.97 12.27,13.22 12.27,9.52 12.92,8.87 P100.72 12.92,8.12
  Top 0.2: D235.P$1 R231.2 28.65,23.25 U230.4
  Top 0.35: 12.92,8.12 v12.92,6.37
  Bottom 0.35: P102.72 v12.92,6.37
PC7  (via drill 0.25)
  Top 0.35: v36.92,13.12 P100.23
  Bottom 0.35: P102.23 v36.92,13.12
PC8  (via drill 0.25)
  Top 0.35: P100.18 v39.92,6.37
  Bottom 0.35: v39.92,6.37 P102.18
PC9  (via drill 0.25)
  Top 0.3: P100.33 v31.92,13.12
  Bottom 0.35: v31.92,13.12 P102.33
PC12  (via drill 0.25)
  Top 0.1: P100.74
  Top 0.35: 11.92,8.37 P100.74 v11.92,6.37
  Bottom 0.35: P102.74 v11.92,6.37
PC14  (via drill 0.25)
  Top 0.35: P100.25 v35.92,13.12
  Bottom 0.35: v35.92,13.12 P102.25
PC15  (via drill 0.25)
  Top 0.35: P100.27 v34.92,13.12
  Bottom 0.35: v34.92,13.12 P102.27
PD6  (via drill 0.25)
  Top 0.35: P100.24 v36.92,6.37
  Bottom 0.35: v36.92,6.37 P102.24
PD7  (via drill 0.25)
  Top 0.35: P100.31 v32.92,13.12
  Bottom 0.35: v32.92,13.12 P102.31
PE7  (via drill 0.25)
  Top 0.35: P100.29 v33.92,13.12
  Bottom 0.35: v33.92,13.12 P102.29
PG9  (via drill 0.25)
  Top 0.1: v10.92,6.37 9.92,5.37 7.42,5.37 5.17,7.62 5.17,12.37 5.71,12.91 EE_WP.TP 6.71,12.91 9.65,15.85 D124.P$1 R108.2 9.55,16.44 9.32,16.67 9.32,17.37 9.17,17.52 U105.P$7
  Top 0.35: P100.76 v10.92,6.37
  Bottom 0.35: P102.76 v10.92,6.37
PG10  (via drill 0.25)
  Top 0.1: v9.92,6.37 9.42,5.87 8.17,5.87 7.92,6.12 7.92,13.37 8.92,14.37 12.42,14.37 20.72,22.67 21.44,22.67 21.44,25.25 23.86,27.67 DEMO_EN1.TP 27.12,27.67 v27.42,27.67 | v31.88,26.61 31.88,23.23 31.32,22.67 30.52,22.67 30.19,23 R202.1
  Top 0.2: U200.B2 30.62,24.07 30.19,23.64 R202.1 29.92,23.37 29.42,23.87 U230.5
  Top 0.35: P100.78 v9.92,6.37
  Bottom 0.1: v27.42,27.67 30.12,27.67 31.12,26.67 31.81,26.67 v31.88,26.61
  Bottom 0.35: v9.92,6.37 P102.78
PG12  (via drill 0.25)
  Top 0.25: 8.92,8.37 P100.80
  Top 0.35: 8.92,8.37 P100.80 v8.92,6.37
  Bottom 0.35: v8.92,6.37 P102.80
PH0  (via drill 0.25)
  Top 0.35: P100.70 v13.92,6.37
  Bottom 0.35: P102.70 v13.92,6.37
POWERGOOD
  Top 0.1: Q121.1 24.31,5.67 U120.2
SENSOR_RAW
  Top 0.1: RT222.1 26.67,25.12
  Top 0.2: U230.1 D223.P$1 RT222.1 | 26.67,25.12 26.92,25.37 C233.1 | C233.1 R224.2 | C225.1 C233.1
  Top 0.25: M220.G1 23.81,18.67 26.32,21.18 26.32,23.67 26.65,24 D223.P$1
TE  (via drill 0.25)
  Top 0.3: P100.35 v30.92,13.12
  Bottom 0.35: v30.92,13.12 P102.35
USB_DN  (via drill 0.25)
  Top 0.1: 9.92,10.9 10.2,10.63 | 10.2,10.63 10.27,10.55 10.27,9.95 v10.12,9.8 | P100.77 9.92,11.52 P100.77 | P100.77 9.92,10.9 | 9.92,10.9 10.2,10.63
  Bottom 0.1: P102.77 9.92,10.75 10.27,10.4 10.27,9.95 v10.12,9.8
USB_DP  (via drill 0.25)
  Top 0.1: P100.75 10.92,10.9 10.57,10.55 10.57,10 v10.77,9.8
  Bottom 0.1: P102.75 10.92,10.75 10.57,10.4 10.57,10 v10.77,9.8
VBUS  (via drill 0.25)
  Top 0.3: P100.11 P102.11
  Top 0.7: P102.11 v42.92,13.62
  Bottom 0.4: P102.11 42.92,12.77
  Bottom 0.8: 42.92,12.77 v42.92,13.12 v42.92,13.62
VSYS  (via drill 0.25)
  Top 0.35: P100.17 v39.92,13.12
  Bottom 0.35: v39.92,13.12 P102.17
(copper drawn outside any net)
  shapes: Bottom circle x12, Top circle x12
